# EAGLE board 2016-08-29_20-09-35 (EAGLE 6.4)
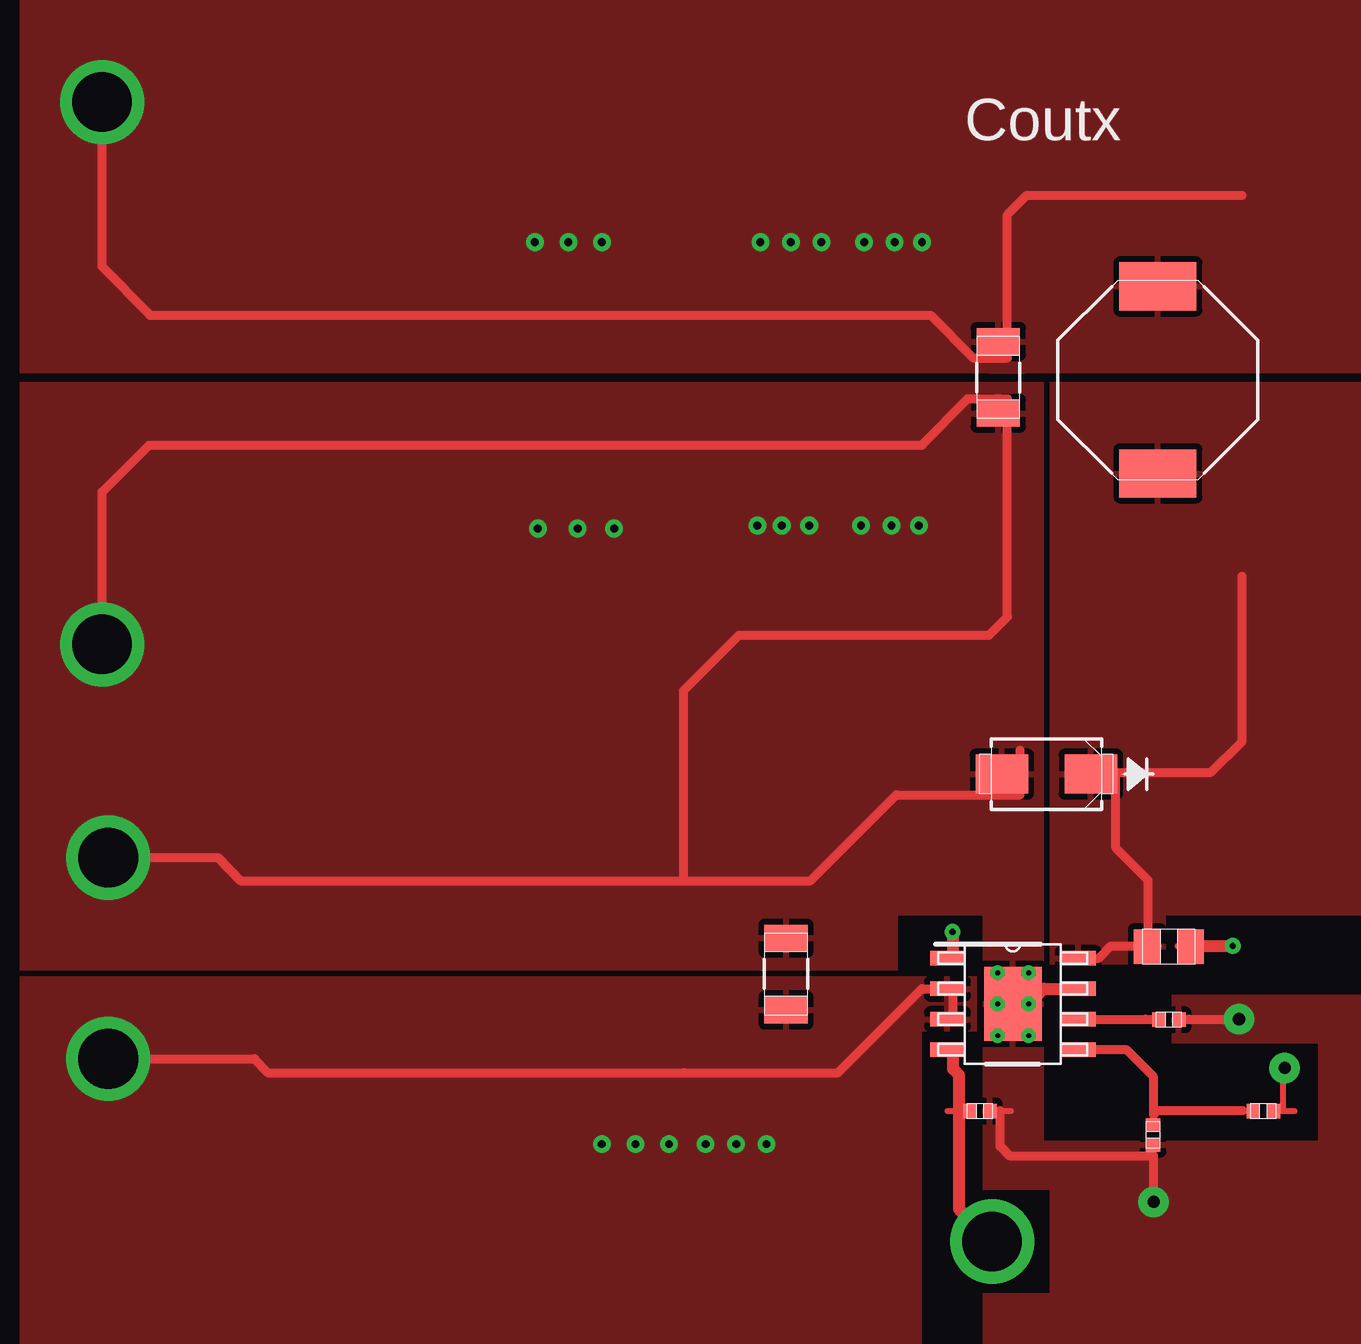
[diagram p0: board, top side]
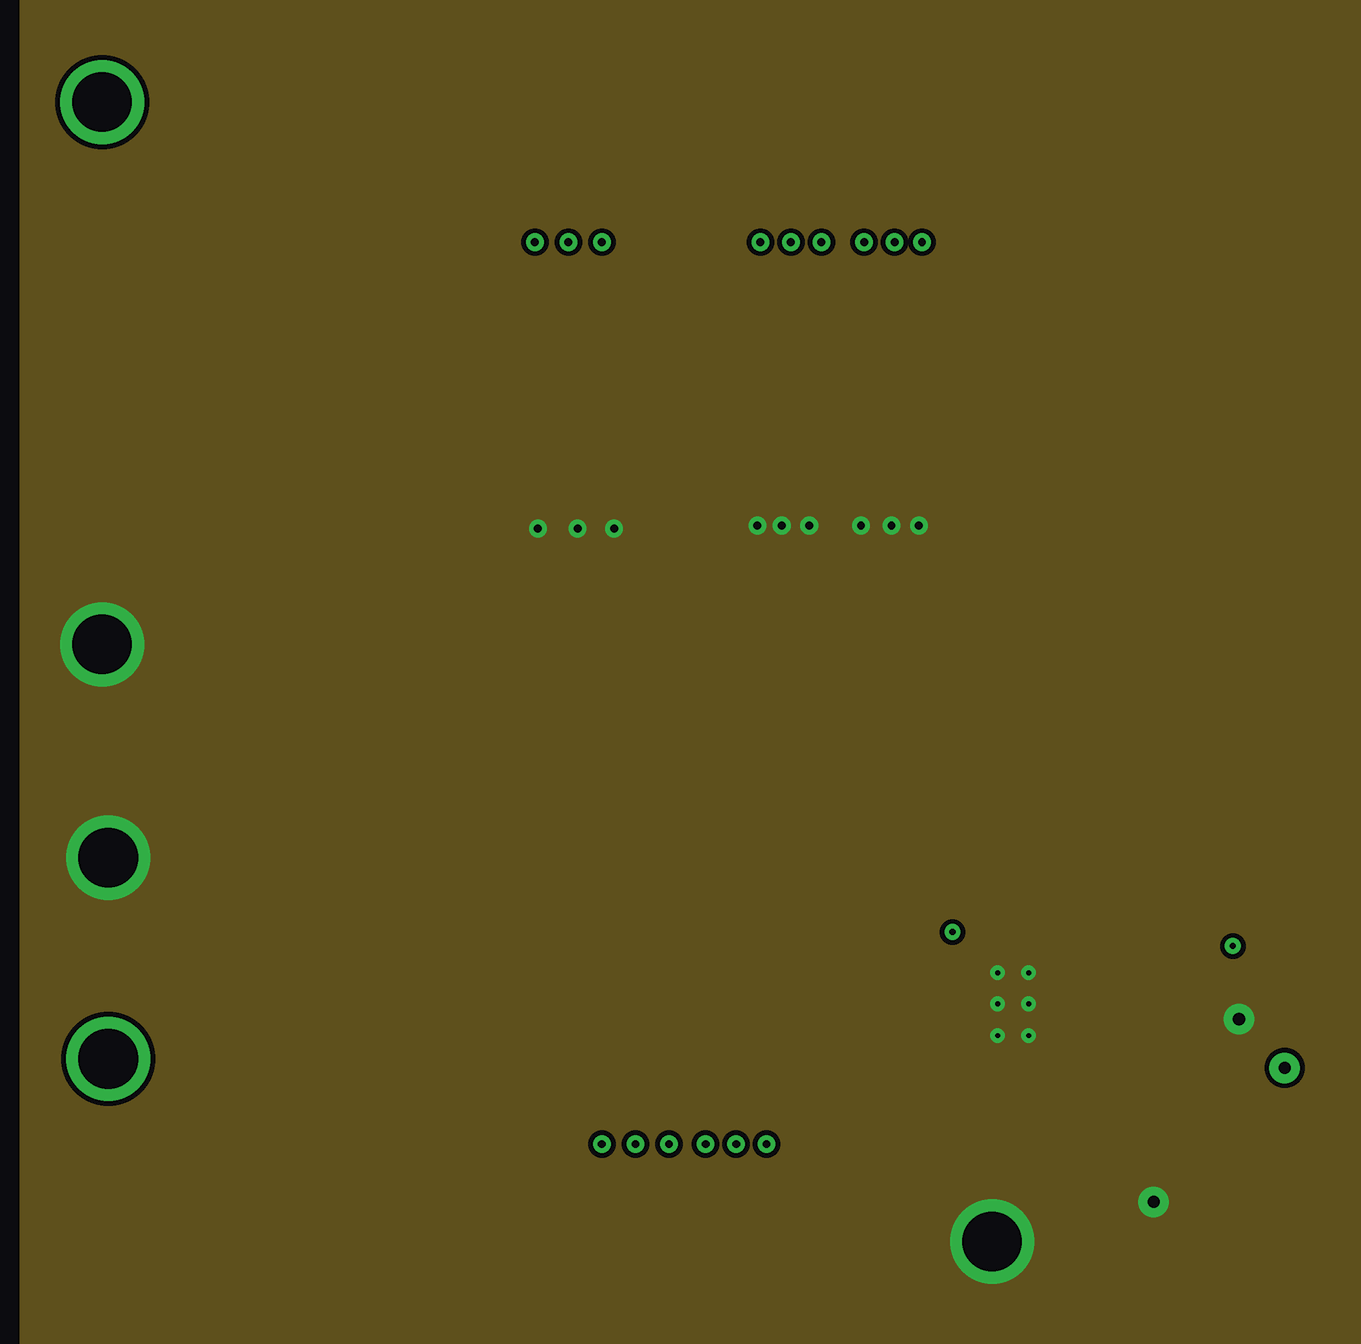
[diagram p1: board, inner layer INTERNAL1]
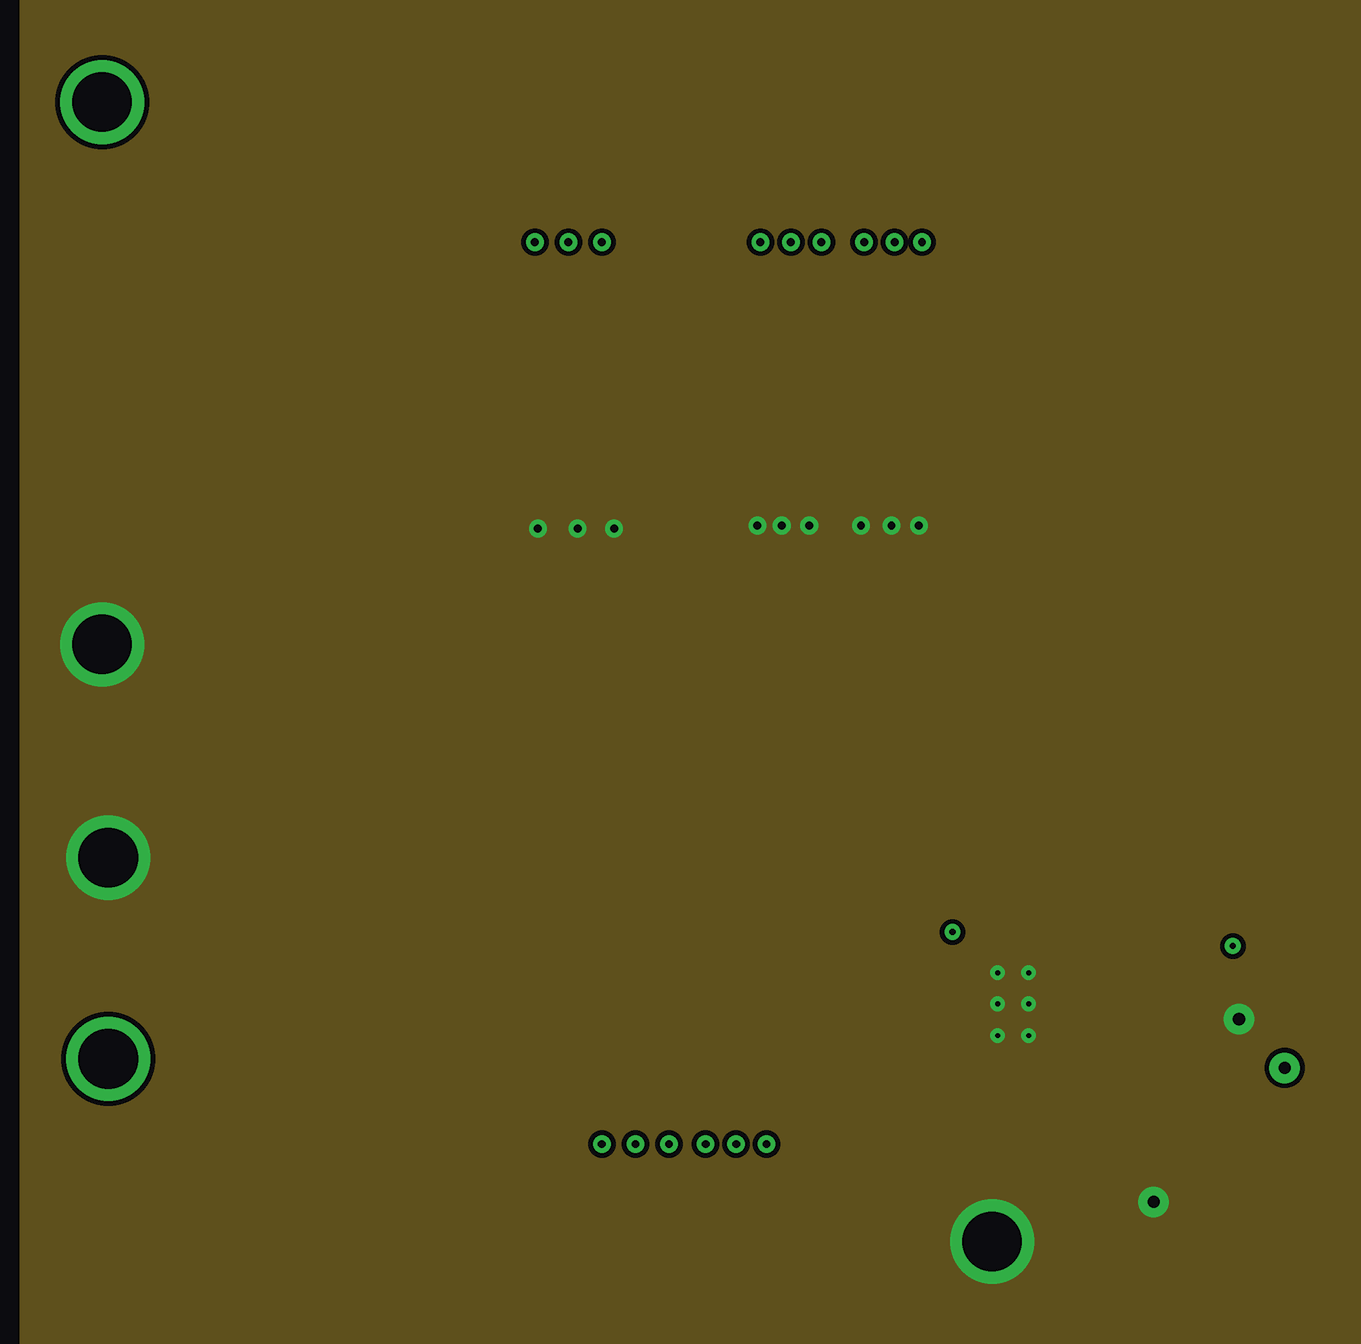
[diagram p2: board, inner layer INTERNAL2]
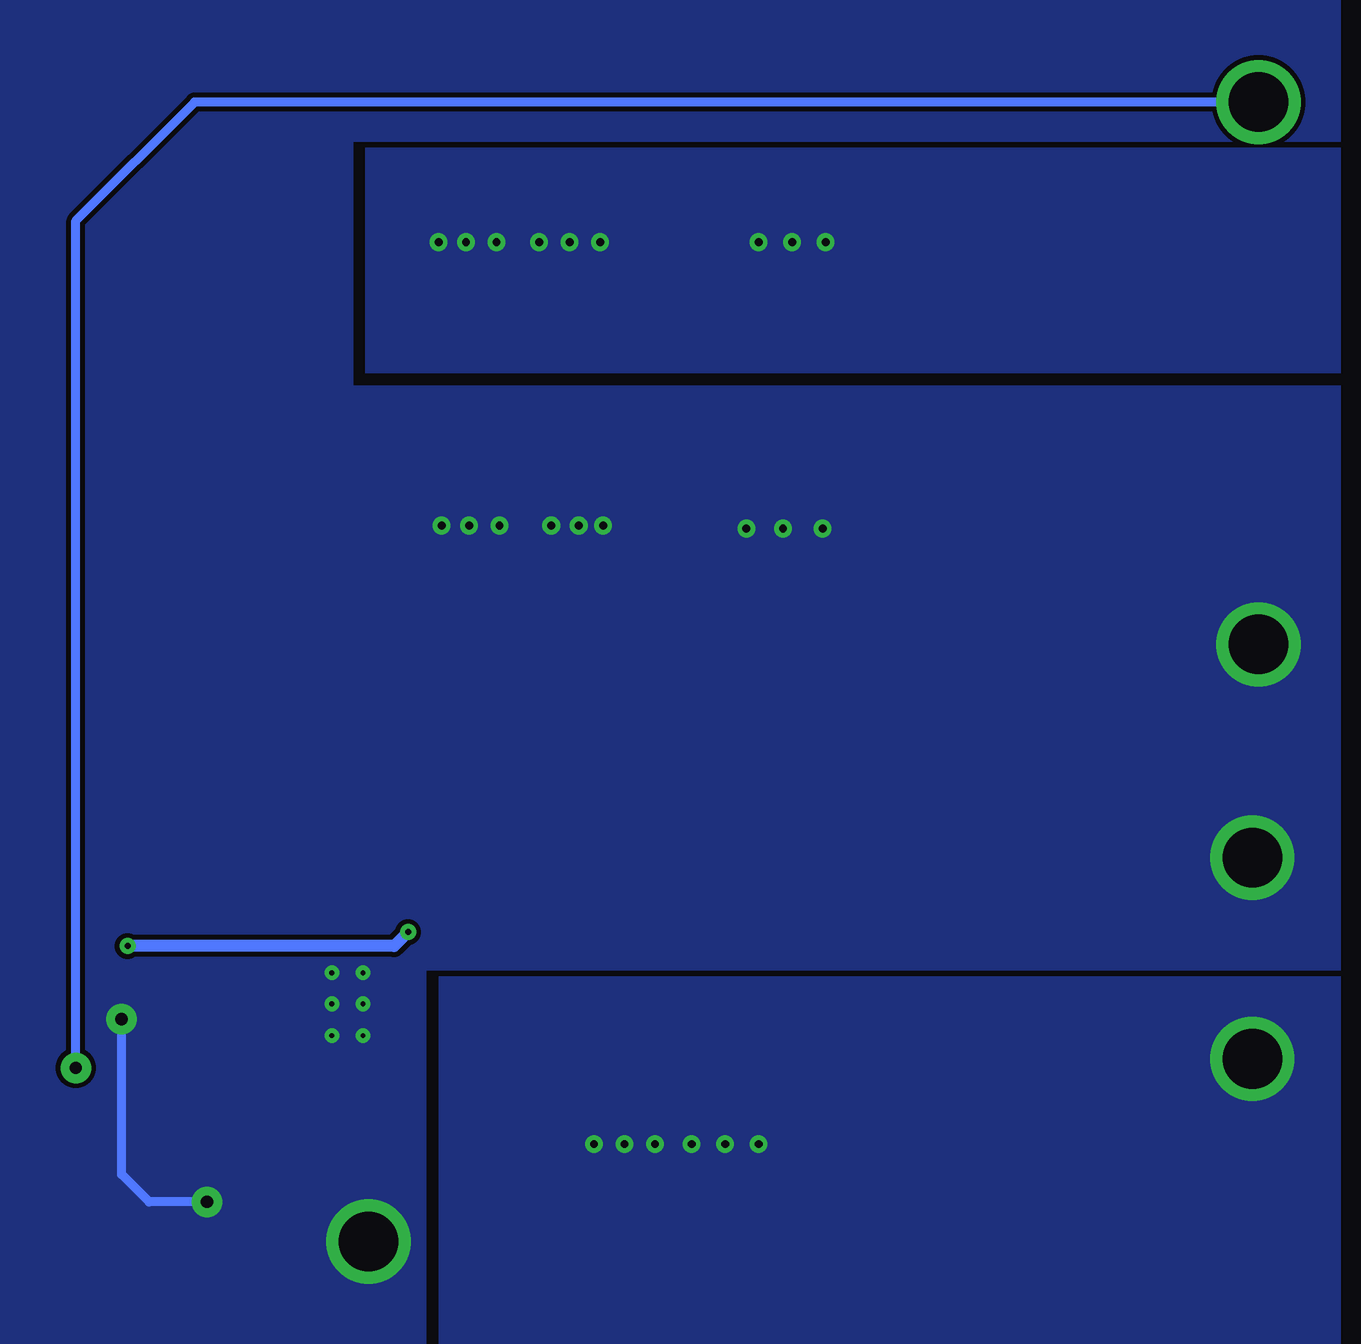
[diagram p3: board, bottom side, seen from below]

No outline drawn. Coordinates in mm, seen from the top.
Copper layers ((1*2)+(15*16)): TOP / INTERNAL1 / layer 15 / BOTTOM

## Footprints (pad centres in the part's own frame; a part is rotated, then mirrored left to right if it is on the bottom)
0805 = smd 1.118 x 1.448: 1 -0.902,0; 2 0.902,0
1206_190 = smd 1.118 x 1.803: 1 -1.499,0; 2 1.499,0
0402 = smd 0.559 x 0.61: 1 -0.419,0; 2 0.419,0
SMA = smd 2.184 x 1.626: 1 -1.854,0; 2 1.854,0
TP-1502 = drill 0.813 round: 1 0,0
SRU8043 = smd 2.007 x 3.2: 1 -3.899,0; 2 3.899,0
DDA0008E_N = smd 1.45 x 0.6: 1 -2.725,1.905; 2 -2.725,0.635; 3 -2.725,-0.635; 4 -2.725,-1.905; 5 2.725,-1.905; 6 2.725,-0.635; 7 2.725,0.635; 8 2.725,1.905 | smd 2.4 x 3.1: 9 0,0

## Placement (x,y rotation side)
Cboot  [0805]  74.55,60.93 180 top
Cin  [1206_190]  58.6,59.79 90 top
Cout  [1206_190]  67.44,84.66 270 top
Css  [0402]  74.55,57.89 0 top
D1  [SMA]  69.44,68.12 180 top
GND  [TP-1502]  30.1,73.51 0 top
GND1  [TP-1502]  30.33,64.62 0 top
L1  [SRU8043]  74.09,84.56 90 top
Rfbb  [0402]  73.89,53.09 270 top
Rfbt  [0402]  78.49,54.08 180 top
Rt  [0402]  66.67,54.08 0 top
U1  [DDA0008E_N]  68.05,58.55 0 top
VIN  [TP-1502]  30.33,56.24 0 top
VOUT  [TP-1502]  30.1,96.11 0 top
VSYNC  [TP-1502]  67.16,48.62 0 top

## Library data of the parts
Cboot = ultra-librarian; RefDes: Cboot; Type: C0805C104K5RACTU
Cin = ultra-librarian; RefDes: Cin; Type: GRM31CR71H225KA88L
Cout = ultra-librarian; RefDes: Cout; Type: GRM31CR61A476KE15L
Css = ultra-librarian; RefDes: Css; Type: GRM155R71C822KA01D
D1 = ultra-librarian; RefDes: D1; Type: B340A-13-F
GND = ultra-librarian; RefDes: GND; Type: TP-1502
GND1 = ultra-librarian; RefDes: GND1; Type: TP-1502
L1 = ultra-librarian; RefDes: L1; Type: SRU8043-3R9Y
Rfbb = ultra-librarian; RefDes: Rfbb; Type: CRCW040210K0FKED
Rfbt = ultra-librarian; RefDes: Rfbt; Type: CRCW040234K0FKED
Rt = ultra-librarian; RefDes: Rt; Type: CRCW040222K1FKED
U1 = ultra-librarian; RefDes: U1; Type: LMR14020SDDAR
VIN = ultra-librarian; RefDes: VIN; Type: TP-1502
VOUT = ultra-librarian; RefDes: VOUT; Type: TP-1502
VSYNC = ultra-librarian; RefDes: VSYNC; Type: TP-1502

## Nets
0: Cin.2 Cout.2 Css.2 D1.2 GND1.1 GND.1 Rfbb.2 Rt.2 U1.7 U1.9
3: Cboot.1 U1.1
4: Rfbb.1 Rfbt.2 U1.5
5: Cboot.2 D1.1 L1.1 U1.8
6: Cout.1 L1.2 Rfbt.1 VOUT.1
7: Css.1 U1.6
11: Cin.1 U1.2 U1.3 VIN.1
14: Rt.1 U1.4 VSYNC.1

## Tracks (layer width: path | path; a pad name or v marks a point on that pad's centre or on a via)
0  (via drill 0.2 pad 0.48, 0.33 pad 0.61, 0.51 pad 1.27, 2.49 pad 3.48)
  TOP 0.254: 67.03,54.09 67.97,54.09 | 73.9,51.74 Rfbb.2 | 74.91,57.9 75.84,57.9
  TOP 0.381: 54.33,63.68 54.33,71.6 56.64,73.91 67.06,73.91 67.82,74.68 67.82,83.77 66.17,83.77 64.26,81.84 62.87,81.84 32.05,81.84 30.1,79.88 v30.1,73.53 | v77.47,57.91 75.39,57.91 74.91,57.91 | v73.91,50.29 73.91,52.22 67.89,52.22 67.51,52.6 67.51,54.1 | 68.35,69.11 68.35,67.26 63.2,67.26 59.61,63.68 54.33,63.68 | v30.35,64.64 34.92,64.64 35.87,63.68 54.33,63.68
  TOP 0.508: v68.71,58.55 69.34,59.18 70.56,59.18
  BOTTOM 0.381: v73.91,50.29 76.33,50.29 77.47,51.44 v77.47,57.91
  other vias: 57.4,78.49 49.91,78.36 51.44,78.36 48.26,78.36 58.42,78.49 59.56,78.49 62.99,78.49 64.14,78.49 61.72,78.49 67.41,58.55 67.41,59.84 67.41,57.23 68.71,57.23 68.71,59.84 67.18,48.64
  pour TOP (rank 5): 26.67,84.45 69.34,84.45 69.34,52.83 80.77,52.83 80.77,56.9 74.68,56.9 74.68,58.93 88.52,58.93 88.52,33.53 26.67,33.53 26.67,43.69 66.8,43.69 66.8,46.48 69.6,46.48 69.6,50.8 66.8,50.8 66.8,62.23 63.25,62.23 63.25,59.94 26.67,59.94
  pour BOTTOM (rank 4): 26.67,84.33 67.82,84.33 67.82,94.49 26.67,94.49 26.67,100.58 100.58,100.58 100.58,26.42 26.67,26.42 26.67,43.69 64.77,43.69 64.77,59.94 26.67,59.94
  pour INTERNAL1 (rank 4): 26.67,100.58 100.58,100.58 100.58,26.42 26.67,26.42
  pour INTERNAL2 (rank 5): 26.67,100.58 26.67,26.42 100.58,26.42 100.58,100.58
3  (via drill 0.25 pad 0.66)
  TOP 0.254: 74.91,60.95 75.84,60.95
  TOP 0.508: v65.53,61.54 65.56,61.49 65.56,60.45 | 75.39,60.96 v77.22,60.96
  BOTTOM 0.508: v77.22,60.96 66.12,60.96 v65.53,61.54
4
  TOP 0.254: 73.9,53.44 73.9,54.38 | 77.14,54.09 Rfbt.2
  TOP 0.381: 77.62,54.1 74.07,54.1 73.91,53.92 73.91,55.5 72.77,56.64 70.56,56.64
5
  TOP 0.254: 73.2,60.95 74.14,60.95
  TOP 0.381: 70.56,60.45 71.63,60.45 72.14,60.96 73.69,60.96 73.69,63.7 72.34,65.05 72.34,68.2 76.3,68.2 77.6,69.49 77.6,76.38
  pour TOP (rank 3): 69.6,84.45 88.65,84.45 88.65,62.23 74.42,62.23 74.42,60.2 69.6,60.2
6  (via drill 0.33 pad 0.61, 0.51 pad 1.27, 2.49 pad 3.48)
  TOP 0.254: 79.32,54.1 79.32,55.83 v79.38,55.88 | 78.84,54.09 79.78,54.09
  TOP 0.381: 77.6,92.25 68.63,92.25 67.82,91.44 67.82,85.47 66.4,85.47 64.62,87.25 62.87,87.25 32.11,87.25 30.1,89.28 v30.1,96.14
  BOTTOM 0.381: v30.1,96.14 74.42,96.14 79.38,91.19 v79.38,55.88
  other vias: 60.07,90.3 49.53,90.3 50.93,90.3 48.13,90.3 58.8,90.3 57.53,90.3 61.85,90.3 63.12,90.3 64.26,90.3
  pour TOP: 67.06,84.81 67.06,86.11 68.55,86.11 68.55,84.81
  pour TOP (rank 2): 26.67,84.84 88.65,84.84 88.65,100.58 26.67,100.58
  pour BOTTOM (rank 2): 26.67,94.23 67.31,94.23 67.31,84.84 26.67,84.84
7
  TOP 0.254: 73.2,57.9 74.14,57.9
  TOP 0.381: 70.56,57.91 73.58,57.91 74.19,57.91
11  (via drill 0.33 pad 0.61, 2.49 pad 3.48)
  TOP 0.381: v30.35,56.26 36.45,56.26 37.01,55.68 54.33,55.68 | 65.56,57.91 65.56,59.18 64.26,59.18 60.76,55.68 54.36,55.68
  other vias: 50.93,52.7 52.32,52.7 53.72,52.7 55.24,52.7 56.52,52.7 57.78,52.7
  pour TOP (rank 3): 66.55,59.69 66.55,57.4 64.26,57.4 64.26,43.94 26.67,43.94 26.67,59.69
  pour BOTTOM: 26.67,59.69 26.67,43.94 64.26,43.94 64.26,59.69
14
  TOP 0.254: 65.33,54.09 Rt.1
  TOP 0.508: 65.56,56.64 65.56,55.83 65.81,55.58 65.81,54.1 65.81,49.99 67.18,48.64

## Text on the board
ASSYNOTES: Coutx | Design Rule: | Min. Clearance: 10mil | Min. Track Width: 10mil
